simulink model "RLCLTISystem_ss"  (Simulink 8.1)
settings: Solver=ode23t  StartTime=0.0  StopTime=100  RelTol=1e-3
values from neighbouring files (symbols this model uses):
  U = 5    [MotorDCParam.m]
undefined symbols (not defined in the file or in its folder): C, L, R
libraries: cstblocks x1

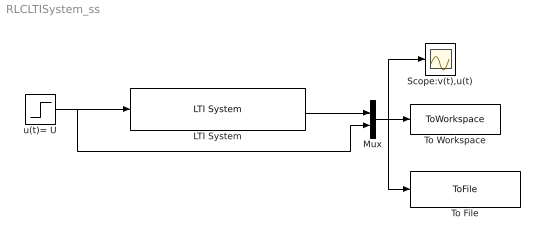
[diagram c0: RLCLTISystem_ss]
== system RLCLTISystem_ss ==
  LTI System : cstblocks/LTI System  sys=ss([0 1/C; -1/L -R/L],[0; 1/L],[1 0],[0])  IC=[ 0;0]
  Mux : Mux  Inputs=2
  Scope:v(t),u(t) : Scope
  To File : ToFile  Filename=RLCLTISystemSS.mat  SaveFormat=Timeseries
  To Workspace : ToWorkspace  VariableName=RLCLTISystemSS  SampleTime=-1
  u(t)= U : Step  Time=0  After=U  SampleTime=0
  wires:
  u(t)= U/1 -> LTI System/1, Mux/2
  LTI System/1 -> Mux/1
  Mux/1 -> To File/1, To Workspace/1, Scope:v(t),u(t)/1
